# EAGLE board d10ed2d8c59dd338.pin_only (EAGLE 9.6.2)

Size 70.36 x 53.34 mm. Coordinates in mm from the lower left corner, seen from the top.
Outline: 0,53.34 0,0 70.36,0 70.36,53.34 0,53.34
Copper layers (1*16): Top 0.035mm / dielectric 1.5mm / Bottom 0.035mm
Design rules "default *": minimum track width 10mil, minimum drill 19mil, track to track 12mil, track to pad 12mil, pad to pad 12mil, via to via 12mil, smd to smd 8mil, copper to edge 20mil, drill to drill 8mil, minimum pad ring 10mil, minimum via ring 8mil, stop-mask expansion 4mil, vias tented up to drill 20mil, thermal gap 10mil

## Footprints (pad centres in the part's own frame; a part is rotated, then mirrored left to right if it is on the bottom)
C0805K = smd 1.1 x 1.4: 1 -1,0; 2 1,0
ILI9325_28INCH_TS = smd 0.5 x 3: 1 -18,27.77; 2 -17,27.77; 3 -16,27.77; 4 -15,27.77; 5 -14,27.77; 6 -13,27.77; 7 -12,27.77; 8 -11,27.77; 9 -10,27.77; 10 -9,27.77; 11 -8,27.77; 12 -7,27.77; 13 -6,27.77; 14 -5,27.77; 15 -4,27.77; 16 -3,27.77; 17 -2,27.77; 18 -1,27.77; 19 0,27.77; 20 1,27.77; 21 2,27.77; 22 3,27.77; 23 4,27.77; 24 5,27.77; 25 6,27.77; 26 7,27.77; 27 8,27.77; 28 9,27.77; 29 10,27.77; 30 11,27.77; 31 12,27.77; 32 13,27.77; 33 14,27.77; 34 15,27.77; 35 16,27.77; 36 17,27.77; 37 18,27.77 | hole 1: -19.5,27; 19.5,27
SO20W = smd 0.66 x 2.032: 1 -5.715,-5.029; 2 -4.445,-5.029; 3 -3.175,-5.029; 4 -1.905,-5.029; 5 -0.635,-5.029; 6 0.635,-5.029; 7 1.905,-5.029; 8 3.175,-5.029; 9 4.445,-5.029; 10 5.715,-5.029; 11 5.715,5.029; 12 4.445,5.029; 13 3.175,5.029; 14 1.905,5.029; 15 0.635,5.029; 16 -0.635,5.029; 17 -1.905,5.029; 18 -3.175,5.029; 19 -4.445,5.029; 20 -5.715,5.029
SOT23-5L = smd 0.55 x 1.2: 1 -0.95,-1.3; 2 0,-1.3; 3 0.95,-1.3; 4 0.95,1.3; 5 -0.95,1.3
SOT23 = smd 1 x 1.4: 1 -0.95,-1.1; 2 0.95,-1.1; 3 0,1.1
SJ = smd 1.168 x 1.6: 1 -0.762,0; 2 0.762,0
SOT23-BEC = smd 1 x 1.4: B -0.95,-1.1; C 0,1.1; E 0.95,-1.1
R0805 = smd 1.3 x 1.5: 1 -0.95,0; 2 0.95,0
ARDUINO-NOHOLE = drill 1 pad 1.676 octagon: 3V 35.56,2.54; 5V 38.1,2.54; A0 50.8,2.54; A1 53.34,2.54; A2 55.88,2.54; A3 58.42,2.54; A4 60.96,2.54; A5 63.5,2.54; AREF 23.876,50.8; D0 63.5,50.8; D1 60.96,50.8; D2 58.42,50.8; D3 55.88,50.8; D4 53.34,50.8; D5 50.8,50.8; D6 48.26,50.8; D7 45.72,50.8; D8 41.656,50.8; D9 39.116,50.8; D10 36.576,50.8; D11 34.036,50.8; D12 31.496,50.8; D13 28.956,50.8; GND 26.416,50.8; GND1 43.18,2.54; GND2 40.64,2.54; RESET 33.02,2.54; VIN 45.72,2.54
MICROSD = smd 0.7 x 1.5: 1 9,-10.64; 2 7.9,-10.24; 3 6.8,-10.64; 4 5.7,-11.04; 5 4.6,-10.64; 6 3.5,-11.04; 7 2.4,-10.64; 8 1.3,-10.64 | smd 1.8 x 1.4: CD1 2,-0.44; CD2 8,-0.44 | smd 1.4 x 1.9: MT1 0.4,-13.54; MT2 13.6,-14.44
FIDUCIAL_1MM = smd 1 x 1: 1 0,0

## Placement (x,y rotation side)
C1  10uF  [C0805K]  19.81,48.51 90 top
C2  0.1uF  [C0805K]  22.61,48.51 90 top
C3  0.1uF  [C0805K]  32,22.86 180 top
C4  0.1uF  [C0805K]  19.05,33.53 90 top
C5  10uF  [C0805K]  30.99,48.51 90 top
CN2  ILI9325_28TFT  [ILI9325_28INCH_TS]  70.1,26.67 270 bottom
IC1  74ACT245DW  [SO20W]  30.73,13.97 270 top
IC3  74ACT245DW  [SO20W]  30.73,38.86 270 top
IC4  ADP122  [SOT23-5L]  26.67,48.51 90 top
IC5  [SOT23]  19.3,41.66 0 top
PIN3  [SJ]  58.67,16.51 270 top
Q1  2222  [SOT23-BEC]  32,26.42 270 top
R1  22  [R0805]  36.83,28.45 0 top
R2  22  [R0805]  36.83,26.42 0 top
R3  22  [R0805]  36.83,24.38 0 top
R4  22  [R0805]  36.83,22.35 0 top
R5  1K  [R0805]  31.75,29.21 180 top
RD  [SJ]  50.29,46.23 90 top
U$2  ARDUINO-NOHOLE  [ARDUINO-NOHOLE]  1.52,53.34 180 bottom
U$3  MICROSD  [MICROSD]  16.76,38.1 270 top
U$7  [ADAFRUIT200MIL]  55.63,28.45 270 top
U$9  [OSHWLOGO_TOL_0.2]  13.97,4.83 0 top
U$10  FIDUCIAL  [FIDUCIAL_1MM]  66.29,46.99 180 top
U$11  FIDUCIAL  [FIDUCIAL_1MM]  4.06,5.08 180 top
VCC  [SJ]  58.67,21.59 270 top

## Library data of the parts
C1-C5 CN2 IC4 IC5 U$2 U$3 U$7 U$9-U$11 = adafruit
IC1 IC3 = 74xx-eu
PIN3 RD VCC = jumper
Q1 = transistor-neu-to92
R1-R5 = rcl

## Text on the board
tPlace: LCD_RD | LCD_WR | LCD_RS | LCD_CS | v1.1 | 2.8" TFT LCD shield | w/Touchscreen | and microSD card | by adafruit! | backlight | D6 | MISO | D4 | LCD_D3 | LCD_D2 | LCD_D1 | LCD_D8 | LCD_D7 | SD_CS | LCD_D5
